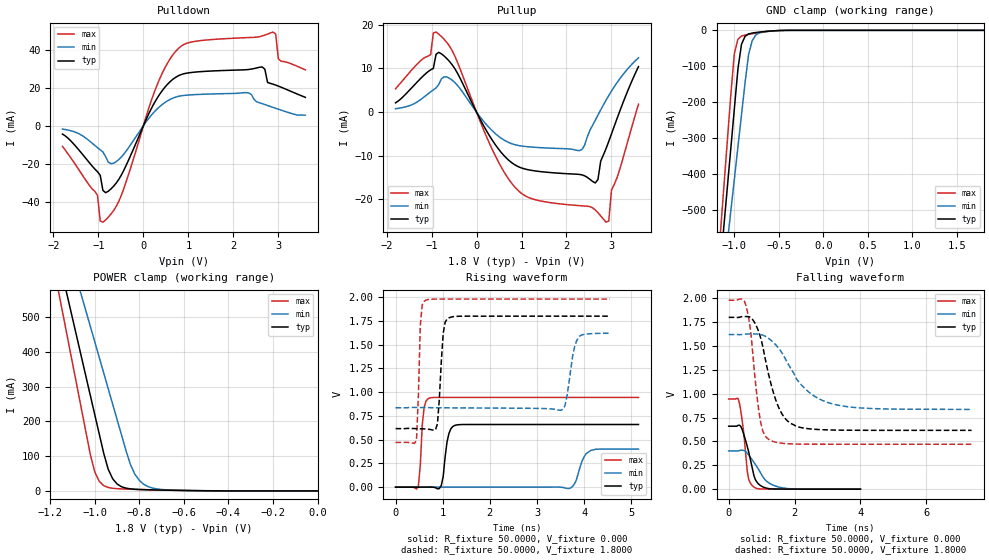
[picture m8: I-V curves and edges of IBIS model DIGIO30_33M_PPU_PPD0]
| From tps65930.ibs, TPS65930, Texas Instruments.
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|   Model DIGIO30_33M_PPU_PPD0
[Model]   DIGIO30_33M_PPU_PPD0
Model_type   I/O
Polarity   Non-Inverting
Enable   Active-Low
Vinl =   0.6900V
Vinh =   1.0500V
Vmeas =   0.9000V
Cref =  30.0000pF
Rref = 100.0000M
Vref =  0.000V
C_comp   30fF   30fF   30fF
[Temperature Range]   25.0000   0.1250k   -40.0000
[Pullup Reference]   1.8000V   1.6200V   1.9800V
[Pulldown Reference]   0.000V   0.000V   0.000V
[POWER Clamp Reference]   1.8000V   1.6200V   1.9800V
[GND Clamp Reference]   0.000V   0.000V   0.000V
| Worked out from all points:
|   slope of the pulldown table from 0 to 0.27 V, typ, clamps not added: 20.7 ohm
|   slope of the pullup table from 0 to 0.27 V, typ, clamps not added: 52.8 ohm
|   GND clamp passes 1 mA (typ) near -0.53 V on its own axis
|   POWER clamp passes 1 mA (typ) near -0.57 V on its own axis
|   rising waveform, R_fixture 50.0000, V_fixture 0.000: 20-80 % time 101ps typ, 163ps min, 71ps max; typ from 0 V to 0.66 V
|   rising waveform, R_fixture 50.0000, V_fixture 1.8000: 20-80 % time 86ps typ, 144ps min, 56.1ps max; typ from 0.616 V to 1.8 V
|   falling waveform, R_fixture 50.0000, V_fixture 0.000: 20-80 % time 278ps typ, 478ps min, 170ps max; typ from 0.66 V to 0 V
|   falling waveform, R_fixture 50.0000, V_fixture 1.8000: 20-80 % time 535ps typ, 981ps min, 280ps max; typ from 1.8 V to 0.616 V
[Pulldown]
| voltage   I(typ)   I(min)   I(max)
-1.8V     -4.367mA   -1.778mA   -10.81mA
-1.02V    -24.17mA   -11.51mA   -36.61mA
-960mV    -26.02mA   -12.66mA   -50.05mA
-900mV    -33.97mA   -13.72mA   -50.66mA
-600mV    -29.98mA   -18.8mA    -42.17mA
300mV     14.24mA    8.688mA    21.12mA
840mV     26.87mA    15.71mA    41.82mA
2.64V     30.88mA    11.61mA    47.13mA
2.88V     21.84mA    9.642mA    49.18mA
2.94V     21.35mA    9.152mA    48.15mA
3V        20.81mA    8.67mA     35.19mA
3.6V      14.89mA    5.551mA    29.32mA
[Pullup]
| voltage   I(typ)   I(min)   I(max)
-1.8V     2.116mA    778.5uA    5.325mA
-1.02V    9.679mA    4.64mA     13.14mA
-900mV    13.23mA    5.525mA    18.33mA
-540mV    10.81mA    7.289mA    14.04mA
300mV     -5.629mA   -3.764mA   -7.458mA
840mV     -12mA      -7.434mA   -17.04mA
2.34V     -14.37mA   -8.6mA     -21.47mA
2.64V     -16.23mA   -1.853mA   -22.42mA
2.88V     -8.337mA   2.739mA    -25.22mA
2.94V     -6.705mA   3.796mA    -24.95mA
3V        -5.002mA   4.808mA    -17.88mA
3.6V      10.42mA    12.43mA    1.793mA
[GND_clamp]
| voltage   I(typ)   I(min)   I(max)
-1.8V     -2.446A    -2.203A    -2.695A
-1.16V    -664.3mA   -773.1mA   -576.5mA
-1.12V    -552.9mA   -683.6mA   -444.3mA
-1.08V    -441.5mA   -594.1mA   -312.4mA
-1.04V    -330.2mA   -504.6mA   -180.8mA
-1V       -219mA     -415.1mA   -65.05mA
-960mV    -108.1mA   -325.6mA   -24.75mA
-920mV    -39.22mA   -236.2mA   -15.92mA
-840mV    -10.11mA   -67.45mA   -11.26mA
-800mV    -7.6mA     -28.85mA   -9.584mA
-720mV    -4.94mA    -7.196mA   -6.432mA
1.8V      135.9pA    840.7nA    181.6pA
[POWER_clamp]
| voltage   I(typ)   I(min)   I(max)
-1.8V     2.435A     2.211A     2.668A
-1.16V    661.6mA    784.7mA    563.4mA
-1.12V    550.8mA    695.5mA    432mA
-1.06V    384.7mA    561.8mA    235.2mA
-1V       218.6mA    428mA      54.19mA
-960mV    108mA      338.9mA    15.18mA
-940mV    62.6mA     294.3mA    9.881mA
-900mV    19.91mA    205.2mA    6.453mA
-840mV    5.873mA    75.72mA    4.919mA
-780mV    3.583mA    18.96mA    3.841mA
-660mV    1.93mA     2.479mA    1.956mA
0V        360.2pA    1.961nA    2.555nA
[Ramp]
| variable   typ   min   max
dV/dt_r   0.3958/0.1489n   0.2403/0.1745n   0.5668/0.5156n
dV/dt_f   0.7102/0.5329n   0.4708/1.0194n   0.9057/0.2903n
R_load = 50.0000
[Rising Waveform]
R_fixture = 50.0000
V_fixture = 0.000
V_fixture_min = 0.000
V_fixture_max = 0.000
| time   V(typ)   V(min)   V(max)
0s        11.15nV    277.6nV    20.93nV
484.8ps   157.4uV    52.86uV    13.34mV
606.1ps   225.8uV    43.4uV     839.2mV
727.3ps   1.084mV    36.73uV    939.3mV
969.7ps   18.1mV     26.86uV    944.7mV
1.131ns   564mV      22.82uV    944.6mV
1.252ns   649.1mV    19.89uV    944.6mV
3.677ns   659.6mV    -14.36mV   944.7mV
4.141ns   659.6mV    387.1mV    944.7mV
5.152ns   659.6mV    400.4mV    944.7mV
[Rising Waveform]
R_fixture = 50.0000
V_fixture = 1.8000
V_fixture_min = 1.6200
V_fixture_max = 1.9800
| time   V(typ)   V(min)   V(max)
0s        616.3mV    835.2mV    470.5mV
444.4ps   616mV      839mV      499.1mV
525.3ps   614.6mV    838.3mV    1.703V
646.5ps   611.7mV    837.4mV    1.969V
888.9ps   668.4mV    836mV      1.98V
1.01ns    1.616V     835.4mV    1.98V
1.091ns   1.77V      835.1mV    1.98V
3.515ns   1.8V       810.5mV    1.98V
3.879ns   1.8V       1.576V     1.98V
4.546ns   1.8V       1.62V      1.98V
[Falling Waveform]
R_fixture = 50.0000
V_fixture = 0.000
V_fixture_min = 0.000
V_fixture_max = 0.000
| time   V(typ)   V(min)   V(max)
0s        659.6mV    400.4mV    944.7mV
282.8ps   668.3mV    399.9mV    950.2mV
323.2ps   670mV      403.5mV    906.7mV
444.4ps   589.7mV    407.2mV    625.7mV
565.7ps   446.3mV    375mV      185.5mV
646.5ps   332.3mV    338.7mV    71.57mV
767.7ps   140.3mV    280.5mV    21.88mV
1.131ns   12.13mV    89.87mV    1.367mV
1.535ns   1.42mV     21.38mV    394.8uV
4ns       9.373uV    120.4uV    4.224uV
[Falling Waveform]
R_fixture = 50.0000
V_fixture = 1.8000
V_fixture_min = 1.6200
V_fixture_max = 1.9800
| time   V(typ)   V(min)   V(max)
0s        1.8V       1.62V      1.98V
525.3ps   1.808V     1.625V     1.922V
646.5ps   1.801V     1.626V     1.708V
848.5ps   1.703V     1.625V     1.006V
969.7ps   1.587V     1.621V     703.2mV
1.252ns   1.145V     1.569V     513.7mV
1.778ns   717.7mV    1.329V     476.7mV
2.303ns   638.7mV    1.058V     471.5mV
2.99ns    621.1mV    910.3mV    470.6mV
7.374ns   616.3mV    835.3mV    470.5mV
